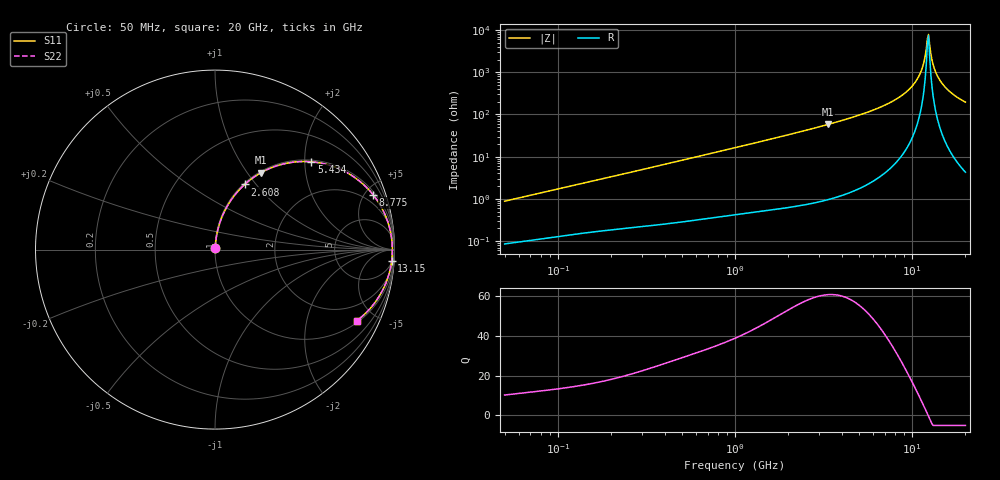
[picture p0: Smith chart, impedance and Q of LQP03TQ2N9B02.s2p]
!Murata Part Number: LQP03TQ2N9B02
!These Parameters are Measured in Series Mode Connection
!  o--[Z]--o
!Port1  Port2
!  o-------o
!Freq. Start=50[MHz] Stop=20[GHz], 401[Steps]
# Hz S RI R 50
!Freq.(Hz) S11(Real) S11(Imag) S21(Real) S21(Imag) S12(Real) S12(Imag) S22(Real) S22(Imag)
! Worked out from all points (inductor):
!   401 points, 50 MHz to 20 GHz, reference 50 ohm
!   read as one part in series: L = 2.77 nH near 51.52 MHz
!   highest Q = 60.6 at 3.364 GHz (marker M1), where L = 2.76 nH
!   self-resonance near 12.2 GHz
!   S11 on the Smith chart (normalised r, x): 50 MHz: 1.00, +0.02; 2.608 GHz: 1.02, +0.88; 5.434 GHz: 1.04, +2.16; 8.775 GHz: 1.22, +5.68; 13.15 GHz: 6, -30; 20 GHz: 1.09, -3.92
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5e7  0.000933 0.00876  0.9991 -0.00876  0.9991 -0.00876  0.000933 0.00876
1.364002e8  0.00205 0.0229  0.998 -0.0229  0.998 -0.0229  0.00205 0.0229
3.721004e8  0.00614 0.0607  0.9939 -0.0607  0.9939 -0.0607  0.00614 0.0607
1e9  0.0297 0.1574  0.9703 -0.1574  0.9703 -0.1574  0.0297 0.1574
2.608132e9  0.1652 0.3629  0.8348 -0.3629  0.8348 -0.3629  0.1652 0.3629
2.728004e9  0.1789 0.3748  0.8211 -0.3748  0.8211 -0.3748  0.1789 0.3748
3.364474e9  0.2569 0.4288  0.7431 -0.4288  0.7431 -0.4288  0.2569 0.4288
5.433528e9  0.5375 0.4892  0.4625 -0.4892  0.4625 -0.4892  0.5375 0.4892
7.442007e9  0.7721 0.4062  0.2279 -0.4062  0.2279 -0.4062  0.7721 0.4062
8.774992e9  0.8809 0.3055  0.1191 -0.3055  0.1191 -0.3055  0.8809 0.3055
9.892087e9  0.9409 0.2092  0.0591 -0.2092  0.0591 -0.2092  0.9409 0.2092
1.082228e10  0.9711 0.1273  0.0289 -0.1273  0.0289 -0.1273  0.9711 0.1273
1.149051e10  0.983 0.0696  0.017 -0.0696  0.017 -0.0696  0.983 0.0696
1.201863e10  0.9874 0.0254  0.0126 -0.0254  0.0126 -0.0254  0.9874 0.0254
1.220001e10  0.988 0.0106  0.012 -0.0106  0.012 -0.0106  0.988 0.0106
1.238412e10  0.9881 -0.00419  0.0119 0.00419  0.0119 0.00419  0.9881 -0.00419
1.257102e10  0.9878 -0.019  0.0122 0.019  0.0122 0.019  0.9878 -0.019
1.314879e10  0.9842 -0.0633  0.0158 0.0633  0.0158 0.0633  0.9842 -0.0633
1.396067e10  0.9733 -0.1213  0.0267 0.1213  0.0267 0.1213  0.9733 -0.1213
1.527346e10  0.9446 -0.204  0.0554 0.204  0.0554 0.204  0.9446 -0.204
1.721783e10  0.886 -0.3018  0.114 0.3018  0.114 0.3018  0.886 -0.3018
2e10  0.7888 -0.3974  0.2112 0.3974  0.2112 0.3974  0.7888 -0.3974
